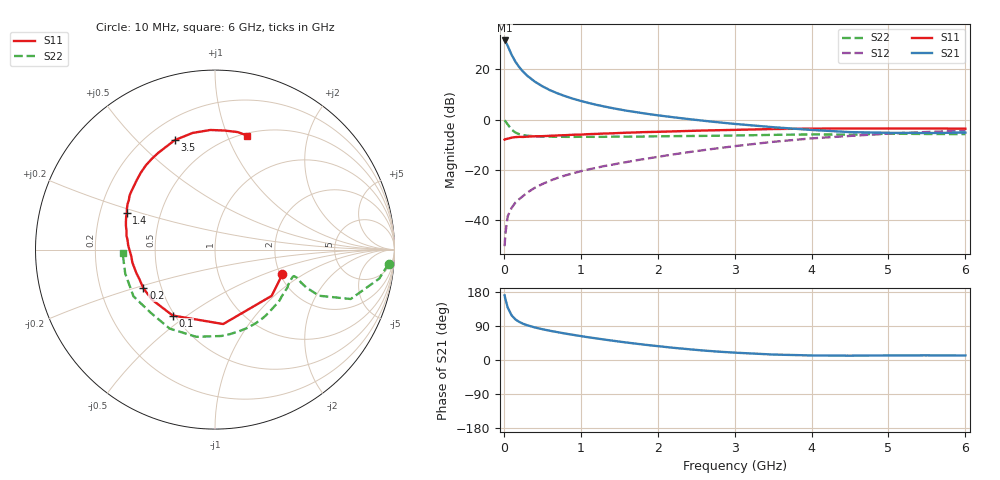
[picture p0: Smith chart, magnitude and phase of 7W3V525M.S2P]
! Infineon Technologies  Discrete & RF Semiconductors
! BFS17W
! Si NPN RF Bipolar Junction Transistor in SOT323
! VCE = 3.5 V  IC = 25 mA
! Common Emitter S-Parameters:  August  1999
# GHz  S  MA  R  50
!  f  S11  S21  S12  S22
! GHz  MAG  ANG  MAG  ANG  MAG  ANG  MAG  ANG
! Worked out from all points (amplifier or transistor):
!   36 points, 10 MHz to 6 GHz, reference 50 ohm
!   highest |S21| = 31.6 dB at 10 MHz (marker M1)
!   |S21| within 3 dB of that: start of sweep to 62.21 MHz
!   unconditionally stable (mu >= 1): 229.3 MHz to 2.246 GHz; 4.632 GHz to end of sweep
!   at 250 MHz: K = 1.04, MAG = 23.5 dB, |S12| = -30.5 dB
!   at 1.4 GHz: K = 1.18, MAG = 8.7 dB, |S12| = -18.0 dB
!   at 6 GHz: K = 1.07, MAG = -2.0 dB, |S12| = -4.4 dB
!   S11 on the Smith chart (normalised r, x): 10 MHz: 2.05, -0.67; 100 MHz: 0.49, -0.44; 200 MHz: 0.40, -0.22; 1.4 GHz: 0.32, +0.18; 3.5 GHz: 0.31, +0.65; 6 GHz: 0.53, +1.18
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0.01  0.3999 -20.1  37.91 170.6  0.003 81.8  0.9703 -4.7
0.02  0.4075 -39.2  36.48 161.0  0.0053 76.1  0.9294 -10.0
0.05  0.4173 -83.7  29.61 138.6  0.0118 65.9  0.8048 -20.0
0.1  0.4364 -122.7  19.81 118.1  0.0173 60.4  0.6343 -23.9
0.15  0.4483 -141.5  14.34 107.1  0.0222 59.7  0.553 -22.6
0.2  0.4536 -151.6  11.14 100.5  0.026 62.3  0.514 -21.0
0.25  0.4521 -158.6  9.049 95.7  0.03 64.0  0.4913 -19.6
0.3  0.4573 -163.5  7.607 92.0  0.0348 65.9  0.4803 -18.9
0.4  0.4659 -171.0  5.768 86.0  0.0435 67.8  0.4653 -18.5
0.5  0.4683 -175.8  4.635 81.3  0.0519 69.5  0.4605 -18.9
0.6  0.4762 -179.6  3.867 77.1  0.0607 70.6  0.4573 -20.0
0.7  0.4842 177.2  3.335 73.4  0.0691 71.5  0.4553 -21.6
0.9  0.4997 170.9  2.61 66.4  0.0853 71.8  0.4524 -25.4
1.1  0.5136 165.1  2.152 59.9  0.1015 71.9  0.4541 -30.0
1.4  0.5325 157.3  1.709 51.4  0.1256 72.6  0.4575 -37.8
1.8  0.5627 147.8  1.35 41.1  0.1616 73.0  0.4601 -49.3
2.2  0.5827 138.5  1.117 32.3  0.2023 72.3  0.469 -61.0
2.8  0.616 124.9  0.881 21.9  0.271 68.9  0.4781 -79.8
3.5  0.6497 110.2  0.707 14.4  0.3612 62.3  0.497 -102.2
4.5  0.667 92.2  0.564 11.4  0.4732 49.0  0.5022 -135.8
5.5  0.6668 79.1  0.54 12.3  0.5673 36.2  0.5176 -165.1
6  0.6602 74.1  0.553 11.9  0.6042 30.0  0.5151 -177.9
